(* Logix 5000 DataType export Banner_ZMX_Data; software revision 33.00 *)

TYPE Banner_ZMX_Data :
STRUCT
   Data_In : Banner_ZMX_Data_In;
   Data_Out : Banner_ZMX_Data_Out;
   Unevenness : INT;
END_STRUCT
END_TYPE

TYPE Banner_ZMX_Data_In :
STRUCT
   Input_Ack : INT;
   Reserved1 : INT;
   Sensor_Fault_Code : INT;
   Boot_Count : INT;   // 1 to 65535
   Up_Time : DINT;   // 1 to 4294967295 in ms
   Missed_Trigger_Count : DINT;
   Reserved2 : INT;
   Reserved3 : INT;
   Reserved4 : INT;
   Reserved5 : INT;
   Reserved6 : INT;
   Reserved7 : INT;
   Reserved8 : INT;
   Reserved30 : INT;
   Frame_Number : DINT;
   Invalid_Pixel_Count : DINT;   // 0 to 56576. Pixels with too little light received to be able to measure.
   Saturated_Pixel_Count : DINT;   // 0 to 56576. Pixels with too much light received to be able to measure.
   Conf_Error_Code : INT;
   Reserved9 : INT;
   Fill_Level_Percent : INT;   // 0 to 200
   Peak_Height : INT;   // 0 to 3500 in mm
   Estimated_Item_Count : INT;
   Output_1_PFM : INT;   // 0. 100 to 600 Hz.
   Output_2_PFM : INT;   // 0. 100 to 600 Hz.
   Trigger_Mode : INT;   // 1 = External, 5 = Internal (uses trigger period), 6 = Free run, 10 = Softa
   Trigger_Period : INT;   // 200 to 60000 ms
   Illumination_Power_Percent : INT;   // 1 to 100
   Reserved10 : INT;
   Reserved11 : INT;
   Reserved12 : INT;
   Reserved13 : INT;
   Reserved14 : INT;
   Reserved15 : INT;
   Reserved16 : INT;
   Reserved17 : INT;
   Pitch_Angle : INT;   // -4500 to 4500 (degrees x 100)
   Roll_Angle : INT;   // -4500 to 4500 (degrees x 100)
   Yaw_Angle : INT;   // -18000 to 18000 (degrees x 100)
   Reserved18 : INT;
   Reserved19 : INT;
   Reserved20 : INT;
   Reserved31 : INT;
   Discrete_IO_Polarity : INT;   // 0 = PNP, 1 = NPN, 2 = Push-Pull
   Reserved21 : INT;
   Fill_Level_Limit_Setpoint_Percent : INT;   // 0 to 200 in mm
   Reserved22 : INT;
   Peak_Height_Limit_Setpoint : INT;   // 0 to 2950 mm
   Reserved23 : INT;
   Discrete_Output_1_Control_Mode : INT;   // 0 = Disabled, 1 = Fill % above setpoint, 2 = Peak height aboe setpoint, 9 = Fill % above setpoint or peak height above setpoint, 10 = Pulse Pro 100 to 600 Hz scaled between 0 to 100%, 11 = Pulse Pro 100 to 600 Hz scaled to peak height above bottom of container, 20 = No output, channle used as input.
   Discrete_Output_2_Control_Mode : INT;   // 0 = Disabled, 1 = Fill % above setpoint, 2 = Peak height aboe setpoint, 9 = Fill % above setpoint or peak height above setpoint, 10 = Pulse Pro 100 to 600 Hz scaled between 0 to 100%, 11 = Pulse Pro 100 to 600 Hz scaled to peak height above bottom of container, 20 = No output, channle used as input.
   ROI_Anchor_Point_X : INT;   // -2500 to 2500
   ROI_Anchor_Point_Y : INT;   // -2500 to 2500
   ROI_Anchor_Point_Z : INT;   // 200 to 3000
   ROI_Length_X : INT;   // 50 to 5000
   ROI_Width_Y : INT;   // 50 to 5000
   ROI_Height_Z : INT;   // 50 to 3000
   Reserved24 : INT;
END_STRUCT
END_TYPE

TYPE Banner_ZMX_Data_Out :
STRUCT
   Control_Bits : INT;
   Reserved1 : INT;
   Trigger_Mode : INT;   // 1 = External, 5 = Internal (uses trigger perdio), 6 = Free Run, 10 = Software
   Trigger_Period : INT;   // 100 to 60000 ms
   Illumination_Power_Precent : INT;   // 0 to 100
   Reserved2 : INT;
   Reserved3 : INT;
   Reserved4 : INT;
   Reserved5 : INT;
   Reserved6 : INT;
   Reserved7 : INT;
   Reserved8 : INT;
   Pitch_Angle : INT;   // -4500 to 4500 (degrees x 100)
   Roll_Angle : INT;   // -4500 to 4500 (degrees x 100)
   Yaw_Angle : INT;   // -18000 to 18000 (degrees x 100)
   Reserved9 : INT;
   Reserved10 : INT;
   Reserved11 : INT;
   Discrete_IO_Polarity : INT;   // 0 = PNP, 1 = NPN, 2 = Push Pull
   Reserved12 : INT;
   Fill_Level_Limit_Setpoint_Percent : INT;   // 0 to 200
   Reserved13 : INT;
   Peak_Height_Limit_Setpoint : INT;   // 0 to 2950 in mm
   Reserved14 : INT;
   Discrete_Output_1_Control_Mode : INT;   // 0 = Disabled, 1 = Fill % above setpoint, 2 = Peak height aboe setpoint, 9 = Fill % above setpoint or peak height above setpoint, 10 = Pulse Pro 100 to 600 Hz scaled between 0 to 100%, 11 = Pulse Pro 100 to 600 Hz scaled to peak height above bottom of container, 20 = No output, channle used as input.
   Discrete_Output_2_Control_Mode : INT;   // 0 = Disabled, 1 = Fill % above setpoint, 2 = Peak height aboe setpoint, 9 = Fill % above setpoint or peak height above setpoint, 10 = Pulse Pro 100 to 600 Hz scaled between 0 to 100%, 11 = Pulse Pro 100 to 600 Hz scaled to peak height above bottom of container, 20 = No output, channle used as input.
   ROI_Anchor_Point_X : INT;   // -2500 to 2500 in mm
   ROI_Anchor_Point_Y : INT;   // -2500 to 2500 in mm
   ROI_Anchor_Point_Z : INT;   // 200 to 3000 in mm
   ROI_Length_X : INT;   // 50 to 5000 in mm
   ROI_Width_Y : INT;   // 50 to 5000 in mm
   ROI_Height_Z : INT;   // 50 to 3000 in mm
   Reserved50 : INT[8];
END_STRUCT
END_TYPE
